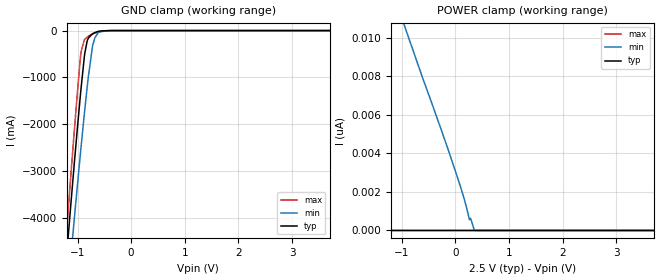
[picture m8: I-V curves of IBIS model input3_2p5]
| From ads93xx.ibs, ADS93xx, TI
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|   input3_2p5 Model
[Model]   input3_2p5
Model_type   Input
Vinl = 0.5
Vinh = 2
|   typ   min   max
C_comp   4.871pF   4.674pF   5.054pF
[Voltage Range]   2.5   2.4   2.6
[Temperature Range]   27   125   -40
[Power Clamp Reference]   2.5   2.4   2.6
[GND Clamp Reference]   0   0   0
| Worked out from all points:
|   GND clamp passes 1 mA (typ) near -0.41 V on its own axis
[GND Clamp]
|   Voltage   I(typ)   I(min)   I(max)
-2.5V     -18.67A    -17.27A    -20.4A
-1.337V   -6.672A    -7.539A    -6.319A
-1.135V   -3.852A    -4.962A    -3.242A
-1.127V   -3.75A     -4.867A    -3.13A
-1.067V   -2.937A    -4.112A    -2.25A
-932.5mV  -1.216A    -2.467A    -445.1mA
-865mV    -487.5mA   -1.694A    -185.3mA
-820mV    -223.2mA   -1.21A     -140.3mA
-722.5mV  -71.54mA   -351.2mA   -71.88mA
-677.5mV  -43.09mA   -158.2mA   -54.18mA
-415mV    -1.147mA   -1.155mA   -2.874mA
5V        0A         0A         0A
[POWER Clamp]
|   Voltage   I(typ)   I(min)   I(max)
-2.5V     1.945nA    116.7nA    498.4pA
-2.485V   0A         48.88nA    0A
-1.488V   0A         14.96nA    0A
-617.5mV  0A         7.988nA    0A
-250mV    0A         5.136nA    0A
35mV      0A         2.802nA    0A
170mV     0A         1.597nA    0A
260mV     0A         591.8pA    0A
282.5mV   0A         633.7pA    0A
350mV     0A         49.06pA    0A
365mV     0A         0A         0A
5V        0A         0A         0A
